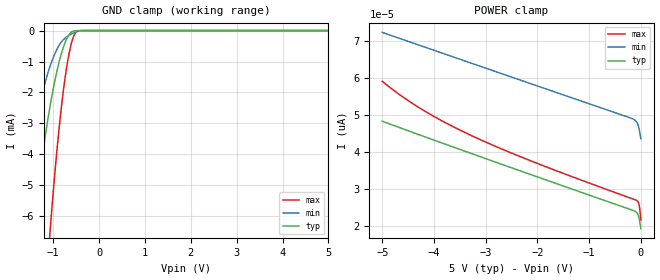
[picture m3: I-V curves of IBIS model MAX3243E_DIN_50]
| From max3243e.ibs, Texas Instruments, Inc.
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[Model]   MAX3243E_DIN_50
Model_type  Input
Vinl=0.8
Vinh=2.4
| variable   typ   min   max
C_comp   2.18pF   1.87pF   2.55pF
[Temperature Range]   40   100   -40
| Ambient temperature   25   85   -40
[Voltage range]   5   4.5   5.5
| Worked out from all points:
|   GND clamp passes 1 mA (typ) near -0.87 V on its own axis
[GND Clamp]
| MAX3243E_DIN_50
|   Voltage   I(typ)   I(min)   I(max)
-5V       -98.57mA   -66.81mA   -159.1mA
-1.81V    -12.1mA    -6.644mA   -25.91mA
-1.43V    -6.37mA    -3.284mA   -14.81mA
-1.255V   -4.27mA    -2.118mA   -10.47mA
-1.085V   -2.588mA   -1.229mA   -6.823mA
-1.065V   -2.415mA   -1.141mA   -6.434mA
-925mV    -1.353mA   -623.4uA   -3.974mA
-805mV    -663.7uA   -335.7uA   -2.265mA
-690mV    -217.6uA   -188.2uA   -1.037mA
-580mV    -27.86uA   -94.61uA   -290uA
-395mV    -43.53nA   -4.739uA   -796.1nA
5V        19.25pA    50.56pA    15.06pA
[POWER Clamp]
| MAX3243E_DIN_50
|   Voltage   I(typ)   I(min)   I(max)
-5V       48.26pA    72.21pA    59.02pA
-4.64V    46.4pA     70.47pA    55.16pA
-4.24V    44.36pA    68.54pA    51.49pA
-3.795V   42.12pA    66.4pA     47.97pA
-3.29V    39.59pA    63.96pA    44.46pA
-2.055V   33.49pA    58.02pA    37.15pA
-205mV    24.44pA    49.14pA    27.52pA
-85mV     23.67pA    48.12pA    26.88pA
-55mV     23.04pA    47.24pA    26.51pA
-35mV     22.15pA    46.22pA    25.76pA
-20mV     21.09pA    45.18pA    24.48pA
-84.45fV  19.25pA    43.55pA    21.55pA
